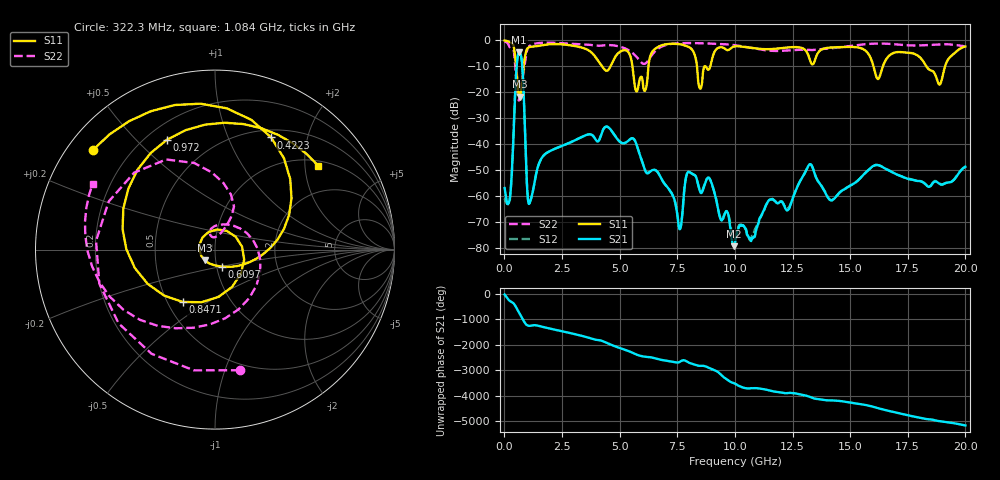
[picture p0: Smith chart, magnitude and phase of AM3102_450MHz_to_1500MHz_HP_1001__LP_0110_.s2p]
!Agilent Technologies,E8364B,MY43040894,A.07.50.67
!Agilent E8364B: A.07.50.67
!Date: Thursday, January 11, 2018 06:02:40
!Correction: S11(Full 2 Port(1,2))
!S21(Full 2 Port(1,2))
!S12(Full 2 Port(1,2))
!S22(Full 2 Port(1,2))
!S2P File: Measurements: S11, S21, S12, S22:
# Hz S  dB  R 50
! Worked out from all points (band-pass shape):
!   1601 points, 10 MHz to 20 GHz, reference 50 ohm
!   highest |S21| = -4.67 dB at 634.7 MHz (marker M1); lowest = -79.4 dB at 9.955 GHz (marker M2)
!   |S21| within 3 dB of the highest: 555.3 MHz to 752.9 MHz (197.6 MHz wide, 30.2 % of centre)
!   lowest |S11| = -21.7 dB at 659.7 MHz (marker M3), VSWR 1.18, Z = 44.3 - j5.27 ohm
!   |S11| at or under -10 dB: 5.555 GHz to 6.248 GHz (693.2 MHz wide, 11.7 % of centre); 16.01 GHz to 16.42 GHz (410.4 MHz wide, 2.53 % of centre); 18.3 GHz to 19.12 GHz (816 MHz wide, 4.36 % of centre)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
!   |S22| runs from -23.2 to -0.4 dB; largest |S21 - S12| = 0.0012
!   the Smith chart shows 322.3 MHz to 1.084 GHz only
!   S11 on the Smith chart (normalised r, x): 322.3 MHz: 0.07, +0.35; 422.3 MHz: 0.59, +1.45; 609.7 MHz: 1.06, -0.20; 847.1 MHz: 0.60, -0.39; 972 MHz: 0.28, +0.62; 1.084 GHz: 1.13, +2.35
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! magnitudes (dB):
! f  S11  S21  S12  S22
! 10 MHz  0.0  -57.0  -61.0  -0.4
! 322.3 MHz  -1.1  -51.3  -51.4  -3.3
! 422.3 MHz  -3.1  -30.0  -29.7  -4.9
! 609.7 MHz  -19.9  -4.9  -4.9  -22.9
! 634.7 MHz  -21.4  -4.7  -4.7  -23.2
! 659.7 MHz  -21.7  -4.8  -4.8  -22.1
! 847.1 MHz  -9.3  -22.8  -22.9  -11.0
! 972 MHz  -3.5  -54.3  -54.1  -4.3
! 1.084 GHz  -2.6  -63.0  -62.7  -2.2
! 3.346 GHz  -2.8  -37.3  -37.3  -1.5
! 5.732 GHz  -19.7  -40.2  -40.1  -6.4
! 6.682 GHz  -2.4  -51.2  -51.2  -3.2
! 7.606 GHz  -1.5  -72.9  -72.5  -1.1
! 7.969 GHz  -2.4  -50.7  -50.8  -1.0
! 8.893 GHz  -10.9  -53.2  -53.2  -1.2
! 9.955 GHz  -2.4  -79.4  -76.7  -1.8
! 10.01 GHz  -2.3  -78.4  -76.3  -1.9
! 13.34 GHz  -9.2  -48.4  -48.4  -3.8
! 14.18 GHz  -2.8  -61.7  -61.7  -3.1
! 16.68 GHz  -6.1  -50.1  -50.1  -1.3
! 18.88 GHz  -17.1  -55.3  -55.3  -1.5
! 20 GHz  -2.4  -48.8  -48.7  -2.3
